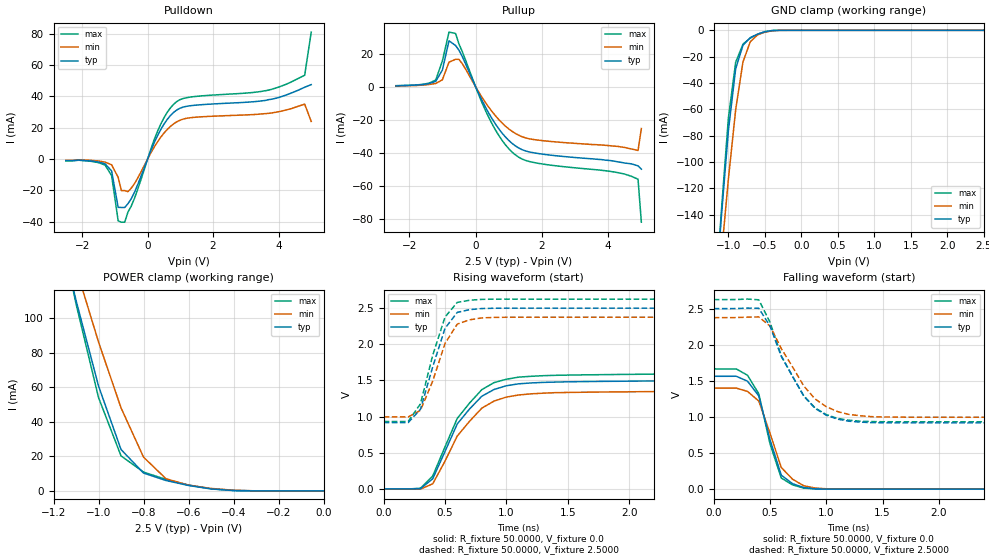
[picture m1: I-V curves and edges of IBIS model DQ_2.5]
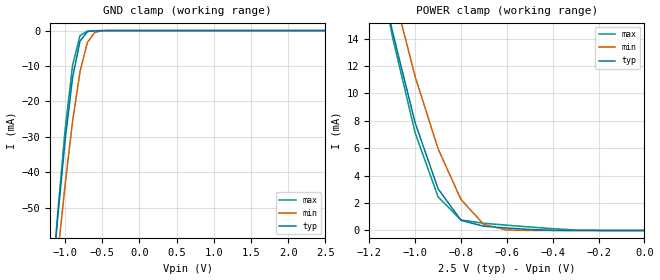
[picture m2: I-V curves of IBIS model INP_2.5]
|*** ISSI Synchronous Sram IBIS Model ***
[IBIS ver]	3.2
[File name]	is61vf204836b100tq.ibs
[File Rev]	1.0
[Date]	May 13,2013
[Notes]
|--- Version History --------------------------------
|1.0: prelimiary
[Disclaimer]	This information is for modeling purpose only
		and is not guaranteed
[Copyright]	INTEGRATED SILICON SOLUTION, INC. 2011
[Component]	IS61VF204836B_100TQ
[Manufacturer]	ISSI
[Package]
| variable   typ   min   max
R_pkg		105.88m			21.330m			174.58m
L_pkg		1.8700nH		0.5900nH		2.5200nH
C_pkg		0.2100pF		0.0600pF		0.2800pF
[Pin]  signal_name   model_name   R_pin   L_pin   C_pin
100   A   INP_2.5
99   A   INP_2.5
98   CEB   INP_2.5
97   CE2   INP_2.5
96   NC   NC
95   NC   NC
94   BWbB   INP_2.5
93   BWaB   INP_2.5
92   CE2B   INP_2.5
91   VDD   POWER
90   VSS   GND
89   CLK   INP_2.5
88   GWB   INP_2.5
87   BWEB   INP_2.5
86   OEB   INP_2.5
85   ADSCB   INP_2.5
84   ADSPB   INP_2.5
83   ADVB   INP_2.5
82   A   INP_2.5
81   A   INP_2.5
80   DQPb   DQ_2.5
79   DQb   DQ_2.5
78   DQb   DQ_2.5
77   VDDQ   POWER
76   VSS   GND
75   DQb   DQ_2.5
74   DQb   DQ_2.5
73   DQb   DQ_2.5
72   DQb   DQ_2.5
71   VSS   GND
70   VDDQ   POWER
69   DQb   DQ_2.5
68   DQb   DQ_2.5
67   VSS   GND
66   NC   NC
65   VDD   POWER
64   ZZ   INP_2.5
63   DQa   DQ_2.5
62   DQa   DQ_2.5
61   VDDQ   POWER
60   VSS   GND
59   DQa   DQ_2.5
58   DQa   DQ_2.5
57   DQa   DQ_2.5
56   DQa   DQ_2.5
55   VSS   GND
54   VDDQ   POWER
53   DQa   DQ_2.5
52   DQa   DQ_2.5
51   DQPa   DQ_2.5
50   A   INP_2.5
49   A   INP_2.5
48   A   INP_2.5
47   A   INP_2.5
46   A   INP_2.5
45   A   INP_2.5
44   A   INP_2.5
43   A   INP_2.5
42   A   INP_2.5
41   VDD   POWER
40   VSS   GND
39   A   INP_2.5
38   A   INP_2.5
37   A0   INP_2.5
36   A1   INP_2.5
35   A   INP_2.5
34   A   INP_2.5
33   A   INP_2.5
32   A   INP_2.5
31   MODE   INP_2.5
30   DQPd   DQ_2.5
29   DQd   DQ_2.5
28   DQd   DQ_2.5
27   VDDQ   POWER
26   VSS   GND
25   DQd   DQ_2.5
24   DQd   DQ_2.5
23   DQd   DQ_2.5
22   DQd   DQ_2.5
21   VSS   GND
20   VDDQ   POWER
19   DQd   DQ_2.5
18   DQd   DQ_2.5
17   VSS   GND
16   NC   NC
15   VDD   POWER
14   NC   NC
13   DQc   DQ_2.5
12   DQc   DQ_2.5
11   VDDQ   POWER
10   VSS   GND
9   DQc   DQ_2.5
8   DQc   DQ_2.5
7   DQc   DQ_2.5
6   DQc   DQ_2.5
5   VSS   GND
4   VDDQ   POWER
3   DQc   DQ_2.5
2   DQc   DQ_2.5
1   DQPc   DQ_2.5
| Models and submodels in the file (2): DQ_2.5 (3-state), INP_2.5 (Input)
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|   Model DQ_2.5
[Model]		DQ_2.5
Model_type	3-state
Polarity   Non-Inverting
Enable   Active-Low
Vmeas = 	0.7500V
Cref = 		5.0000pF
Rref = 		50.0000
Vref = 		1.2500V
C_comp   3.8290pF   3.3420pF   4.0300pF|
[Temperature Range]	  25.0000   100.0000   0.0
[Voltage Range]   2.5000V   2.3750V   2.6250V
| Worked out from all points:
|   slope of the pulldown table from 0 to 0.375 V, typ, clamps not added: 21.1 ohm
|   slope of the pullup table from 0 to 0.375 V, typ, clamps not added: 24.7 ohm
|   GND clamp passes 1 mA (typ) near -0.49 V on its own axis
|   POWER clamp passes 1 mA (typ) near -0.48 V on its own axis
|   rising waveform, R_fixture 50.0000, V_fixture 0.0: 20-80 % time 314ps typ, 320ps min, 316ps max; typ from 0 V to 1.51 V
|   rising waveform, R_fixture 50.0000, V_fixture 2.5000: 20-80 % time 170ps typ, 187ps min, 169ps max; typ from 0.918 V to 2.5 V
|   falling waveform, R_fixture 50.0000, V_fixture 0.0: 20-80 % time 169ps typ, 190ps min, 167ps max; typ from 1.56 V to 0 V
|   falling waveform, R_fixture 50.0000, V_fixture 2.5000: 20-80 % time 314ps typ, 336ps min, 308ps max; typ from 2.5 V to 0.918 V
[Pulldown]
|Voltage	  I(typ)   I(min)   I(max)
-2.5V     -1mA       -900uA     -1.1mA
-1.3V     -3.1mA     -1.98mA    -3.85mA
-1.1V     -7.6mA     -3.69mA    -10.56mA
-900mV    -30.82mA   -11.68mA   -39.46mA
-800mV    -30.93mA   -20.13mA   -40.31mA
-700mV    -30.93mA   -20.13mA   -40.31mA
-400mV    -21.21mA   -15.69mA   -25.04mA
300mV     14.77mA    10.9mA     17.5mA
800mV     29.84mA    22.52mA    35.05mA
3.7V      37.9mA     29.16mA    43.99mA
4.8V      45.8mA     35.01mA    53.46mA
5V        47.5mA     23.97mA    81.01mA
[Pullup]
|Voltage	  I(typ)   I(min)   I(max)
-2.4V     400uA      360uA      550uA
-1.2V     3.2mA      1.89mA     3.96mA
-1V       9.97mA     4.104mA    15.48mA
-800mV    27.74mA    14.77mA    33.01mA
-600mV    24.84mA    16.54mA    32.14mA
-400mV    18.24mA    13.88mA    21.25mA
300mV     -12.46mA   -9.666mA   -14.47mA
1V        -32.57mA   -25.6mA    -37.58mA
1.6V      -39.48mA   -31.55mA   -45.26mA
4.1V      -44.9mA    -35.91mA   -51.48mA
4.9V      -48mA      -38.7mA    -56.1mA
5V        -50mA      -25.39mA   -82.14mA
[GND_clamp]
|Voltage	  I(typ)   I(min)   I(max)
-2.5V     -1.238A    -1.081A    -1.377A
-1.2V     -220.2mA   -237.3mA   -225.5mA
-1.1V     -144.4mA   -173.5mA   -140.5mA
-1V       -76.37mA   -113.2mA   -66.76mA
-900mV    -29.2mA    -60.35mA   -24.24mA
-800mV    -11.34mA   -23.99mA   -10.52mA
-700mV    -5.573mA   -8.7mA     -5.892mA
-600mV    -2.907mA   -3.457mA   -3.011mA
-500mV    -1.075mA   -1.408mA   -999.8uA
-300mV    -9.492uA   -41.34uA   -5.052uA
2.5V      40.97nA    416.1nA    43nA
[POWER_clamp]
|Voltage	  I(typ)   I(min)   I(max)
-2.5V     946.2mA    803.1mA    1.061A
-1.2V     165.2mA    174.2mA    170.3mA
-1.1V     110.4mA    129mA      108.4mA
-1V       60.76mA    86.26mA    54.07mA
-900mV    23.99mA    48.12mA    20.31mA
-800mV    10.36mA    19.57mA    10.92mA
-700mV    6.025mA    7.051mA    6.647mA
-600mV    3.142mA    3.321mA    3.423mA
-500mV    1.147mA    1.448mA    1.242mA
-400mV    194.4uA    400.6uA    266.4uA
0V        40.97nA    40.9nA     75.05nA
[Ramp]
| variable   typ   min   max
dV/dt_r		0.9042/0.2795n   0.7824/0.2922n   0.9954/0.2697n
dV/dt_f		0.9493/0.2827n   0.8275/0.2702n   1.0156/0.3061n
R_load =	50.0000
[Rising Waveform]
R_fixture=	50.0000
V_fixture=	0.0
V_fixture_min=	0.0
V_fixture_max=	0.0
|time   V(typ)   V(min)   V(max)
0s        0V         0V         0V
300ps     3.703mV    -2.782mV   10.28mV
400ps     140.9mV    71.68mV    179.8mV
600ps     899.4mV    732.5mV    975.4mV
800ps     1.282V     1.117V     1.373V
900ps     1.375V     1.216V     1.47V
1ns       1.427V     1.27V      1.516V
1.2ns     1.466V     1.315V     1.557V
1.6ns     1.484V     1.337V     1.577V
5ns       1.507V     1.359V     1.602V
[Rising Waveform]
R_fixture=	50.0000
V_fixture=	2.5000
V_fixture_min=	2.3750
V_fixture_max=	2.6250
|time   V(typ)   V(min)   V(max)
0s        917.8mV    995.8mV    932.4mV
200ps     917.8mV    995.8mV    932.6mV
300ps     1.101V     1.087V     1.177V
400ps     1.689V     1.492V     1.849V
500ps     2.221V     2.011V     2.377V
600ps     2.441V     2.279V     2.579V
700ps     2.478V     2.338V     2.608V
800ps     2.494V     2.365V     2.621V
900ps     2.498V     2.372V     2.623V
5ns       2.5V       2.375V     2.625V
[Falling Waveform]
R_fixture=	50.0000
V_fixture=	0.0
V_fixture_min=	0.0
V_fixture_max=	0.0
|time   V(typ)   V(min)   V(max)
0s        1.563V     1.4V       1.665V
200ps     1.563V     1.399V     1.665V
300ps     1.495V     1.353V     1.577V
400ps     1.292V     1.22V      1.321V
500ps     684mV      773.4mV    627.2mV
600ps     194.2mV    300.3mV    154.3mV
700ps     76.23mV    138.2mV    59.74mV
800ps     22.14mV    46.86mV    14.45mV
1.1ns     594.5uV    1.764mV    405.6uV
5ns       23.76uV    34.03uV    20.31uV
[Falling Waveform]
R_fixture=	50.0000
V_fixture=	2.5000
V_fixture_min=	2.3750
V_fixture_max=	2.6250
|time   V(typ)   V(min)   V(max)
0s        2.5V       2.375V     2.625V
400ps     2.505V     2.385V     2.622V
500ps     2.259V     2.258V     2.31V
600ps     1.839V     1.948V     1.847V
800ps     1.289V     1.429V     1.292V
900ps     1.119V     1.25V      1.126V
1ns       1.024V     1.142V     1.033V
1.1ns     969.7mV    1.075V     979.6mV
1.5ns     919.4mV    999.8mV    933.8mV
5ns       917.8mV    995.8mV    932.4mV
|   Model INP_2.5
[Model]		INP_2.5
Model_type	Input
Polarity   Non-Inverting
Enable   Active-Low
Vinl = 		0.8000V
Vinh = 		2.0000V
C_comp   3.8290pF   3.3420pF   4.0300pF|
[Temperature Range]	  25.0000   100.0000   0.0
[Voltage Range]   2.5000V   2.3750V   2.6250V
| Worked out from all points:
|   GND clamp passes 1 mA (typ) near -0.73 V on its own axis
|   POWER clamp passes 1 mA (typ) near -0.81 V on its own axis
[GND_clamp]
|Voltage	  I(typ)   I(min)   I(max)
-2.5V     -434.7mA   -399mA     -475.2mA
-1.2V     -76.89mA   -84.89mA   -78.19mA
-1.1V     -52.83mA   -63.46mA   -51.66mA
-1V       -30.98mA   -43.42mA   -27.92mA
-900mV    -13.28mA   -25.61mA   -9.811mA
-800mV    -2.971mA   -11.61mA   -1.401mA
-700mV    -287uA     -3.303mA   -148.3uA
-600mV    -52.18uA   -480.7uA   -48.72uA
-500mV    -11.21uA   -45.78uA   -9.079uA
2.5V      40.19nA    40.4nA     42.61nA
[POWER_clamp]
|Voltage	  I(typ)   I(min)   I(max)
-2.5V     189.7mA    171.9mA    207.8mA
-1.2V     22.77mA    25.28mA    23.03mA
-1.1V     14.57mA    17.73mA    14.18mA
-1V       7.84mA     11.21mA    7.108mA
-900mV    3.038mA    5.954mA    2.453mA
-800mV    736uA      2.255mA    762.7uA
-700mV    308.2uA    432.8uA    524.6uA
-600mV    181.1uA    36.29uA    386.3uA
-400mV    10.09uA    187.6nA    130.9uA
-300mV    415nA      89.24nA    33.9uA
0V        40.19nA    23.22nA    74.57nA
